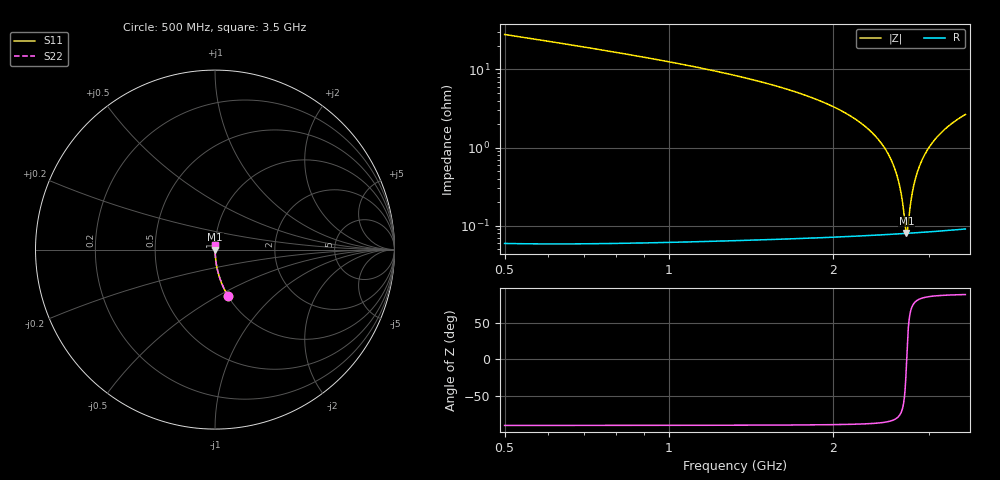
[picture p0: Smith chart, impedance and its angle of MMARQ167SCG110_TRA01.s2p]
! MMARQ167SCG110_TRA01  S-PARAMETER MODEL  ( General Type )
! Model Generated by TAIYO YUDEN Corporation (http://www.ty-top.com)
! Version 1.0
! TAIYO YUDEN Control No. 160201
! Copyright(c) 2016 TAIYO YUDEN CO.,LTD. All Rights Reserved.
! Product Description (link to TY-COMPAS)
! https://ds.yuden.co.jp/TYCOMPAS/or/detail?pn=MMARQ167SCG110JTRA01&u=M
! Products Name : Multilayer Ceramic Capacitors
! Characteristics :
!  Capacitance : 11 pF , Rated Voltage : 250V , TCC : CG / C0G
!  Case Size : 1.6 x 0.8 / 0.063 x 0.031 [mm/inch] , Thickness : 0.7 / 0.028 [mm/inch]
!  (Conditions: Temperature = 25 degC , DC Bias Current/Voltage = 0A / 0V)
! External Node Assignments :
!  1  o---| |---o  2
! GND o---------o GND
! Frequency Range : 500MHz  -  3500MHz  [ 401 STEP ]
# MHz S RI R 50
! Freq[MHz].  S11 Real  S11 Imag  S21 Real  S21 Imag  S12 Real  S12 Imag  S22 Real  S22 Imag
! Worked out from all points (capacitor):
!   401 points, 500 MHz to 3.5 GHz, reference 50 ohm
!   read as one part in series: C = 11 pF near 515 MHz
!   lowest |Z| = 81.2 mohm at 2.728 GHz (marker M1)
!   series resonance near 2.731 GHz, so ESL is about 310 pH
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500  0.0731 -0.2592  0.9269 0.2592  0.9269 0.2592  0.0731 -0.2592
725  0.0338 -0.1792  0.9662 0.1792  0.9662 0.1792  0.0338 -0.1792
1002.5  0.0159 -0.1228  0.9841 0.1228  0.9841 0.1228  0.0159 -0.1228
1505  0.00512 -0.0666  0.9949 0.0666  0.9949 0.0666  0.00512 -0.0666
2000  0.00184 -0.0335  0.9982 0.0335  0.9982 0.0335  0.00184 -0.0335
2300  0.00108 -0.0183  0.9989 0.0183  0.9989 0.0183  0.00108 -0.0183
2412.5  0.000933 -0.0132  0.9991 0.0132  0.9991 0.0132  0.000933 -0.0132
2502.5  0.000857 -0.00926  0.9991 0.00926  0.9991 0.00926  0.000857 -0.00926
2577.5  0.000818 -0.00613  0.9992 0.00613  0.9992 0.00613  0.000818 -0.00613
2637.5  0.000801 -0.00369  0.9992 0.00369  0.9992 0.00369  0.000801 -0.00369
2675  0.000797 -0.0022  0.9992 0.0022  0.9992 0.0022  0.000797 -0.0022
2712.5  0.000798 -0.000723  0.9992 0.000723  0.9992 0.000723  0.000798 -0.000723
2727.5  0.000799 -0.000139  0.9992 0.000139  0.9992 0.000139  0.000799 -0.000139
2742.5  0.000801 0.000441  0.9992 -0.000441  0.9992 -0.000441  0.000801 0.000441
2787.5  0.000812 0.00216  0.9992 -0.00216  0.9992 -0.00216  0.000812 0.00216
2810  0.000819 0.00301  0.9992 -0.00301  0.9992 -0.00301  0.000819 0.00301
2840  0.000831 0.00414  0.9992 -0.00414  0.9992 -0.00414  0.000831 0.00414
2907.5  0.000867 0.00662  0.9991 -0.00662  0.9991 -0.00662  0.000867 0.00662
3005  0.000939 0.0101  0.9991 -0.0101  0.9991 -0.0101  0.000939 0.0101
3102.5  0.00103 0.0135  0.999 -0.0135  0.999 -0.0135  0.00103 0.0135
3215  0.00117 0.0173  0.9988 -0.0173  0.9988 -0.0173  0.00117 0.0173
3500  0.00161 0.0265  0.9984 -0.0265  0.9984 -0.0265  0.00161 0.0265
